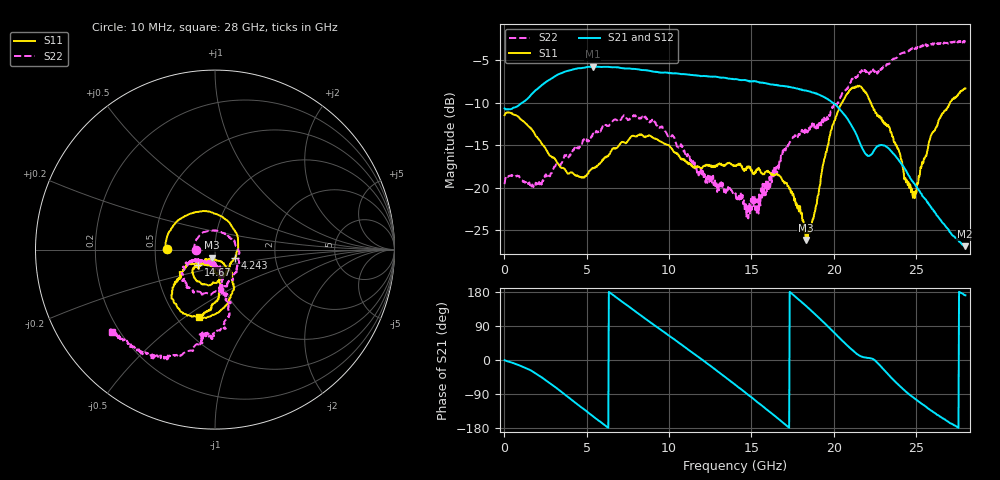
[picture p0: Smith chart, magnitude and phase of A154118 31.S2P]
!  2-Port S-parameters saved by WinCal
! VAR MeasName=S-Parameters (CALIBRATED_DATA) read from VNA (N5230A)
! VAR MeasDate=2015-9-10 14:36:42
! VAR NAME=A154118 31
! VAR FILENAME=A154118 31.S2P
! VAR DATE=2015-9-10 14:36:42
! VAR PHYS_PORTS=1,2
# Hz S DB R 50
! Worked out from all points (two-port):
!   801 points, 10 MHz to 28 GHz, reference 50 ohm
!   highest |S21| = -5.73 dB at 5.363 GHz (marker M1); lowest = -26.9 dB at 27.97 GHz (marker M2)
!   |S21| within 3 dB of the highest: 1.77 GHz to 18.64 GHz (16.87 GHz wide, 165 % of centre)
!   lowest |S11| = -26.2 dB at 18.31 GHz (marker M3), VSWR 1.10, Z = 48 - j4.37 ohm
!   |S11| at or under -10 dB: start of sweep to 20.5 GHz; 22.27 GHz to 27.07 GHz (4.798 GHz wide, 19.5 % of centre)
!   |S22| runs from -23.6 to -2.6 dB; largest |S21 - S12| = 0.0081
!   S11 on the Smith chart (normalised r, x): 10 MHz: 0.58, +0.00; 4.243 GHz: 1.24, -0.12; 14.67 GHz: 0.82, -0.14; 28 GHz: 0.65, -0.57
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1e7  -11.44 179.8  -10.65 -0.4  -10.71 -0.3  -19.59 -179.1
1.199575e9  -12.27 125.2  -9.83 -19.5  -9.85 -19.3  -19.25 101.5
2.354162e9  -15.05 69.1  -7.78 -48.5  -7.78 -48.3  -19.23 31.1
4.243488e9  -18.47 -22.7  -6.03 -110.4  -6.00 -110.4  -15.35 -45.6
4.698325e9  -18.76 -39.1  -5.91 -125.8  -5.88 -125.9  -14.87 -56.3
5.363088e9  -17.67 -52.3  -5.73 -148.0  -5.71 -148.0  -13.65 -71.2
6.972512e9  -14.97 -85.6  -5.86 159.2  -5.81 159.0  -12.15 -100.0
9.351662e9  -14.40 -128.3  -6.41 84.2  -6.37 84.0  -12.84 -141.9
1.173081e10  -17.46 -136.4  -6.80 9.4  -6.73 8.8  -17.98 -154.4
1.4005e10  -17.40 -134.8  -7.22 -64.8  -7.19 -65.3  -20.82 -133.7
1.466976e10  -17.94 -138.0  -7.33 -87.4  -7.28 -87.8  -21.98 -112.4
1.662906e10  -18.56 -135.3  -7.92 -154.8  -7.90 -155.5  -17.38 -72.4
1.830846e10  -26.18 -112.1  -8.56 143.1  -8.55 142.9  -13.44 -78.5
1.869332e10  -24.00 -78.9  -8.77 128.2  -8.80 127.7  -12.42 -81.5
1.98829e10  -13.10 -62.6  -9.91 78.7  -9.89 77.8  -10.82 -78.1
2.093252e10  -8.61 -93.6  -12.18 34.0  -12.14 33.1  -8.05 -81.3
2.194716e10  -8.76 -131.5  -16.03 6.4  -16.04 5.3  -6.39 -92.8
2.334666e10  -12.88 -146.0  -15.39 -40.0  -15.39 -40.9  -5.41 -99.8
2.488611e10  -20.83 -101.8  -19.49 -100.2  -19.61 -100.5  -3.48 -113.5
2.593574e10  -13.77 -79.6  -22.33 -134.0  -22.44 -134.2  -3.13 -124.9
2.796501e10  -8.29 -103.2  -26.91 170.9  -26.93 170.8  -2.71 -142.6
2.8e10  -8.31 -103.1  -26.90 170.7  -27.00 170.0  -2.64 -141.3
